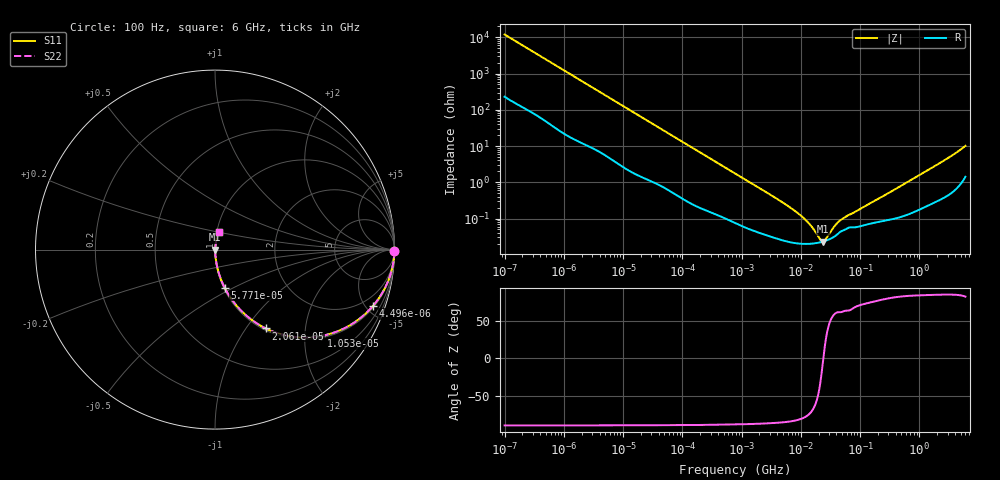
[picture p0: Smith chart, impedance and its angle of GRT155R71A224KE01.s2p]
!Murata Part Number: GRT155R71A224KE01
!These Parameters are Measured in Series Mode Connection
!Data Generated on Jun 19, 2026
!  o--ll--o
!Port1  Port2
!  o------o
!Operation Temp=25[degC], DC Bias Voltage=0[V]
!Freq. Start=100[Hz] Stop=6[GHz] 401[Steps]
# Hz S RI R 50
!Freq.(Hz) S11(Real) S11(Imag) S21(Real) S21(Imag) S12(Real) S12(Imag) S22(Real) S22(Imag)
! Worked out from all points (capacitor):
!   401 points, 100 Hz to 6 GHz, reference 50 ohm
!   read as one part in series: C = 132 nF near 109 Hz
!   lowest |Z| = 23.2 mohm at 23.28 MHz (marker M1)
!   series resonance near 24 MHz, so ESL is about 330 pH
!   S11 on the Smith chart (normalised r, x): 100 Hz: open; 4.496 kHz: 1.12, -5.58; 10.53 kHz: 1.05, -2.41; 20.61 kHz: 1.03, -1.24; 57.71 kHz: 1.01, -0.45; 6 GHz: 1.03, +0.20
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100  0.9998 -0.00834  0.000229 0.00834  0.000229 0.00834  0.9998 -0.00834
600  0.9967 -0.0487  0.0033 0.0487  0.0033 0.0487  0.9967 -0.0487
2008  0.9715 -0.1568  0.0285 0.1568  0.0285 0.1568  0.9715 -0.1568
4496  0.881 -0.313  0.119 0.313  0.119 0.313  0.881 -0.313
6728  0.7741 -0.4076  0.2259 0.4076  0.2259 0.4076  0.7741 -0.4076
10527  0.5908 -0.4815  0.4092 0.4815  0.4092 0.4815  0.5908 -0.4815
20606  0.2824 -0.4391  0.7176 0.4391  0.7176 0.4391  0.2824 -0.4391
40335  0.0993 -0.2862  0.9007 0.2862  0.9007 0.2862  0.0993 -0.2862
57709  0.0536 -0.2121  0.9464 0.2121  0.9464 0.2121  0.0536 -0.2121
169018  0.00825 -0.0774  0.9918 0.0774  0.9918 0.0774  0.00825 -0.0774
774597  0.00106 -0.0176  0.9989 0.0176  0.9989 0.0176  0.00106 -0.0176
6644369  0.000225 -0.00199  0.9998 0.00199  0.9998 0.00199  0.000225 -0.00199
1.087309e7  0.000201 -0.00105  0.9998 0.00105  0.9998 0.00105  0.000201 -0.00105
1.555665e7  0.000203 -0.000535  0.9998 0.000535  0.9998 0.000535  0.000203 -0.000535
2.128304e7  0.00022 -0.000143  0.9998 0.000143  0.9998 0.000143  0.00022 -0.000143
2.327686e7  0.000229 -3.62e-05  0.9998 3.62e-05  0.9998 3.62e-05  0.000229 -3.62e-05
2.662322e7  0.000246 0.000123  0.9998 -0.000123  0.9998 -0.000123  0.000246 0.000123
3.64232e7  0.000313 0.000503  0.9997 -0.000503  0.9997 -0.000503  0.000313 0.000503
4.764863e7  0.000443 0.000807  0.9996 -0.000807  0.9996 -0.000807  0.000443 0.000807
3.124326e8  0.000943 0.0051  0.9991 -0.0051  0.9991 -0.0051  0.000943 0.0051
2.048624e9  0.00399 0.0309  0.996 -0.0309  0.996 -0.0309  0.00399 0.0309
6e9  0.0234 0.0963  0.9766 -0.0963  0.9766 -0.0963  0.0234 0.0963
